PROGRAM MAIN
VAR 
	i 			: INT;
	fbRead		: ARRAY[0..2] OF Default_NN_Read;
	nOut		: ARRAY[0..2] OF array[0..10 ] of INT;
	iState		: ARRAY[0..2] OF INT;
	bError		: ARRAY[0..2] OF BOOL;
	bBusy		: ARRAY[0..2] OF BOOL;
	nErrorID	: ARRAY[0..2] OF DWORD;
	Finish_Reading	: ARRAY[0..2] OF BOOL;
	
	ServerUrl	: STRING(MAX_STRING_LENGTH) := 'opc.tcp://192.168.0.2:4840';
	NameSpaceUri: STRING(MAX_STRING_LENGTH) := 'urn:CX-121E6A:BeckhoffAutomation:Ua:PLC1';
	NodeIdentifier	: ARRAY[0..2] OF STRING(MAX_STRING_LENGTH)	:= ['MAIN.structure_test.a', 'MAIN.iter2','MAIN.iteration3'];
END_VAR


	(*i := i + 1;
	IF i = 3 THEN
		i := 0;
	END_IF*)
	FOR i := 0 TO 2 BY 1 DO
		

	fbRead[i](
		ServerUrl_IN			:= ServerUrl,
		NameSpaceUri_IN			:= NameSpaceUri,
		NodeIdentifier_IN		:= NodeIdentifier[i],
		FinishReadingSignal_IN	:= Finish_Reading[i],
		iState_OUT				=> iState[i],
		Error_OUT				=> bError[i],
		Busy_OUT				=> bBusy[i],
		ErrorID_OUT				=> nErrorID[i],
		ReadingOntheNode_OUT	=> nOut[i]
	);
	END_FOR

END_PROGRAM
